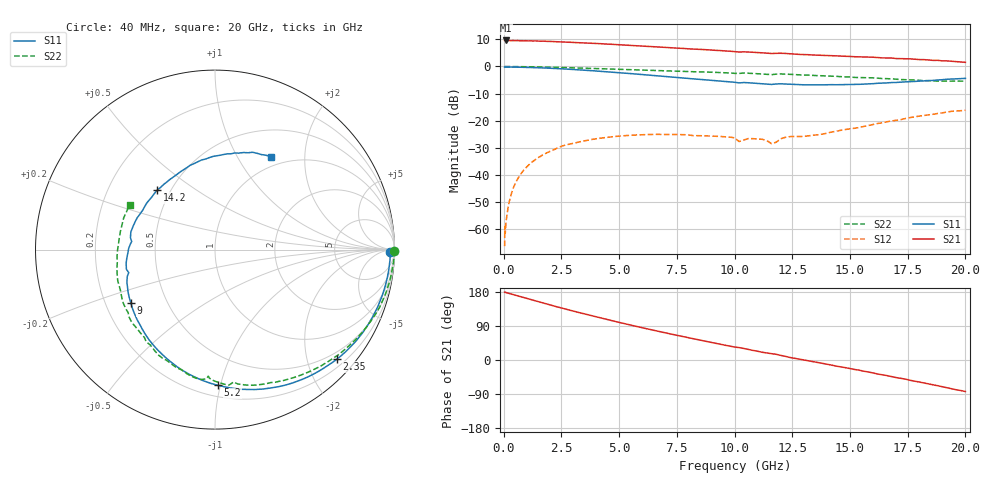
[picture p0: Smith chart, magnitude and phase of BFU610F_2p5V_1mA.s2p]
! Filename:  P:\Prog\Test\Noise\ATS_data\Testdata_Net\SplitFiles\BFU610_2W_A5_HighFreq_2.5V_1mA_D.s2p
! Date/Time: Wed 10/Aug/2011 16:55:05
! BFU610_2W_A5_HighFreq_Bias1_2.5V_1mA_10mA_R.s2p
! MDIF S-parameter v. bias file
! BFU610_2W_A5_HighFreq_2.5V_1mA_10mA
! Date/time Mon Aug 08 14:04:20 2011
! bias mode 1
! bias variable = I_out
! VAR bias_var= 1
! VAR V_out= 2.5010
! VAR I_out= 0.9950
! VAR V_in= 0.8484
! VAR I_in= 0.0073
! Device data file deembeded for feedlines and parallel
! Original file: \SplitFiles\BFU610_2W_A5_HighFreq_2.5V_1mA_R.s2p
! Feed-files: PR003V01_101208_Feed1.s2p, PR003V01_101208_Feed2.s2p
! Parallel-file: PR003V01_101208_Par.s2p
# MHz S MA R 50
!  Freq-MHz  S11-mag  S11-arg  S21-mag  S21-arg  S12-mag  S12-arg  S22-mag  S22-arg
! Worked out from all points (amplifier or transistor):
!   167 points, 40 MHz to 20 GHz, reference 50 ohm
!   highest |S21| = 9.6 dB at 80 MHz (marker M1)
!   |S21| within 3 dB of that: start of sweep to 7.873 GHz
!   unconditionally stable (mu >= 1): 7.813 GHz to end of sweep
!   at 550 MHz: K = -0.01, MSG = 26.0 dB, |S12| = -42.4 dB
!   at 4.2 GHz: K = 0.41, MSG = 17.4 dB, |S12| = -26.4 dB
!   at 20 GHz: K = 1.12, MAG = 6.7 dB, |S12| = -16.1 dB
!   S11 on the Smith chart (normalised r, x): 40 MHz: 67, -36; 2.35 GHz: 0.35, -2.58; 5.2 GHz: 0.28, -0.98; 9 GHz: 0.31, -0.27; 14.2 GHz: 0.42, +0.36; 20 GHz: 0.86, +1.40
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40  0.977 -0.7  3.02 179.2  0.0004831 85.4  0.9977 -0.4
50  0.9697 -1.2  3.009 179.3  0.001132 86.3  0.9979 -0.5
60  0.9765 -0.8  3.013 178.4  0.0008326 77.3  0.9983 -0.6
80  0.9766 -1.4  3.023 178.4  0.001001 91.2  0.9983 -0.8
140  0.9766 -2.5  3.008 177.4  0.001812 91.8  0.9981 -1.4
280  0.9752 -5.0  3.005 174.9  0.003784 90.5  0.9975 -2.8
700  0.9692 -12.6  2.986 167.6  0.009795 83.9  0.9935 -6.9
1350  0.9527 -24.2  2.968 156.4  0.01884 74.2  0.9836 -13.2
2350  0.9133 -41.8  2.867 139.7  0.032 61.8  0.9608 -22.6
3400  0.8605 -59.5  2.73 123.1  0.04167 48.0  0.933 -31.8
4300  0.8101 -74.3  2.622 109.5  0.04819 38.2  0.9074 -39.2
5200  0.7565 -88.7  2.489 96.5  0.0527 29.5  0.8809 -46.3
6800  0.6644 -113.8  2.275 74.3  0.0558 15.9  0.8371 -58.4
9000  0.5554 -147.4  2.011 46.4  0.05198 5.2  0.7842 -74.5
10200  0.4974 -165.1  1.847 32.7  0.04125 -1.5  0.7444 -82.0
11600  0.4664 174.4  1.736 16.7  0.03756 7.4  0.7063 -93.0
12000  0.479 168.2  1.755 12.2  0.04635 22.3  0.7281 -96.2
13400  0.4605 145.8  1.63 -4.5  0.05402 20.6  0.6846 -110.0
14200  0.462 134.1  1.586 -13.4  0.0617 24.1  0.667 -118.1
16800  0.5051 98.4  1.434 -43.8  0.09892 17.7  0.5913 -150.0
18400  0.549 78.6  1.32 -63.4  0.1282 5.8  0.5473 -175.9
20000  0.6043 58.9  1.193 -83.2  0.1558 -10.4  0.5367 152.4
